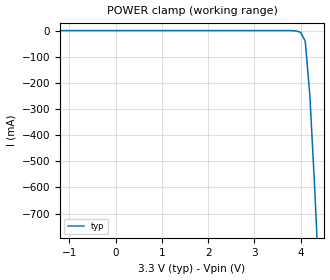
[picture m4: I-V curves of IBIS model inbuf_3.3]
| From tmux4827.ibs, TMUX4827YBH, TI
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|   Voltage   I(typ)   I(min)   I(max)
| inbuf_3.3
[Model]   inbuf_3.3
Model_type   Input
Vinl = 0.8
Vinh = 1.2
|   typ   min   max
C_comp   2.533030e-12   NA   NA
[Voltage Range]   3.3   NA   NA
[Temperature Range]   27   NA   NA
[Power Clamp Reference]   3.3   NA   NA
[GND Clamp Reference]   0   NA   NA
[GND Clamp]
|   Voltage   I(typ)   I(min)   I(max)
[POWER Clamp]
|   Voltage   I(typ)   I(min)   I(max)
-3.3V     142.6nA    NA         NA
3.7V      -5.997uA   NA         NA
3.9V      -1.496mA   NA         NA
4V        -6.748mA   NA         NA
4.1V      -40.59mA   NA         NA
4.2V      -249.6mA   NA         NA
4.3V      -588mA     NA         NA
4.4V      -968.4mA   NA         NA
6.6V      -6.329A    NA         NA
